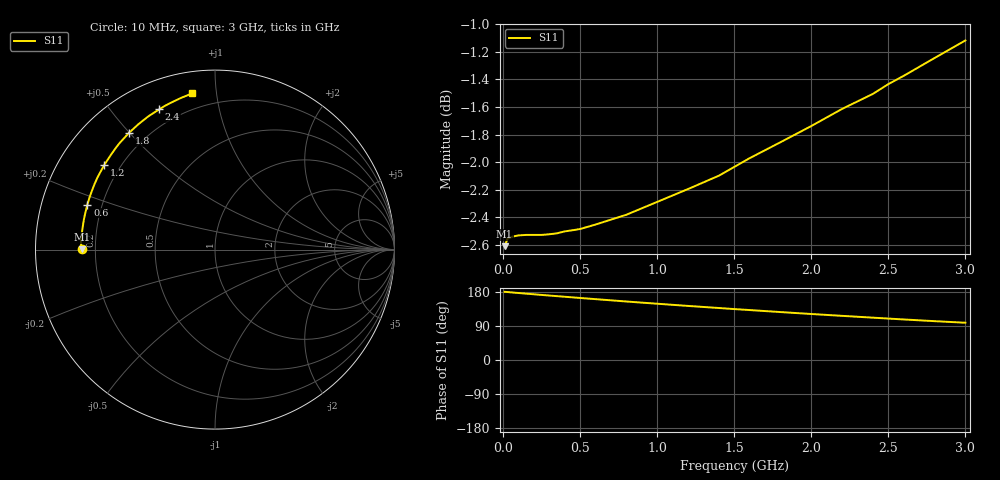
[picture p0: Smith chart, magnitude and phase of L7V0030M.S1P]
! SIEMENS Small Signal Semiconductors
! BAR14-1
! Si PIN Diode in SOT23
! IF = 30 mA
! S-Parameters:  July  1992
# GHz  S  MA  R  50
!  f  S11
! GHz  MAG  ANG
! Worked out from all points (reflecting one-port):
!   31 points, 10 MHz to 3 GHz, reference 50 ohm
!   lowest |S11| = -2.6 dB at 10 MHz (marker M1), VSWR 6.70, Z = 7.46 + j0.0427 ohm
!   phase of S11 starts at 180 deg and turns -82 deg over the sweep
!   S11 on the Smith chart (normalised r, x): 10 MHz: 0.15, +0.00; 600 MHz: 0.14, +0.17; 1.2 GHz: 0.14, +0.33; 1.8 GHz: 0.13, +0.50; 2.4 GHz: 0.13, +0.67; 3 GHz: 0.11, +0.86
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0.01  0.7404 179.9
0.03  0.7452 179.3
0.05  0.7458 178.6
0.06  0.7463 178.2
0.1  0.7471 176.8
0.15  0.7474 175.1
0.2  0.7474 173.4
0.25  0.7474 171.7
0.35  0.7484 168.5
0.4  0.7496 166.9
0.5  0.7511 163.7
0.6  0.7539 160.6
0.7  0.757 157.5
0.8  0.7601 154.4
0.9  0.7642 151.4
1  0.7683 148.5
1.2  0.7766 142.7
1.4  0.7853 137.2
1.5  0.7911 134.4
1.6  0.7969 131.8
1.8  0.8076 126.5
2  0.8186 121.4
2.2  0.8304 116.5
2.4  0.8409 111.7
2.5  0.8478 109.3
2.6  0.8537 107.0
2.8  0.8665 102.5
3  0.8793 98.3
